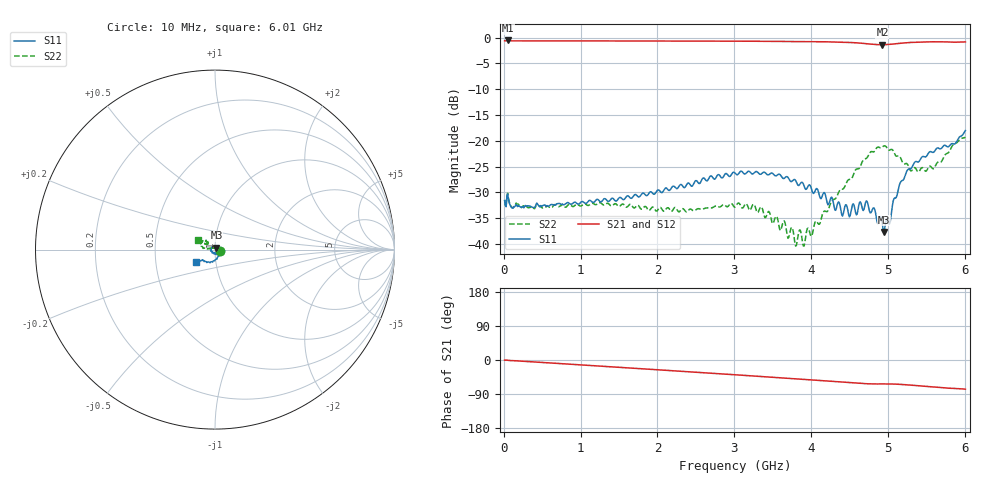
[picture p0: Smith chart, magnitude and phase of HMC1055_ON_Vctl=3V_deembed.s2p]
! Device:	HMC1055
! Description:	GaAs MMIC SPST Switch
! Package:	LP2 8 pin 2x2 mm QFN Plastic Package
! Frequency:	0.5 -  4 GHz
! Ports:
! RF1 = Port 1
! RF2 = Port 2
! State: ON
! Supply Votage: Vdd = 3 V
! ControlVoltage: Vctl = 3 V
! Data:	Data was collected using a calibrated network analyzer with AFR software.
!	Fixtures were calculated using AFR and fixturing was applied to collect
!	this Deembedded  S Parameter data of HMC1055.
!  The reference plane is the edge of the package pin.
! Note:	Analog Devices supplies this data as a sample of measured data at the package pin
!	for this product.  Your particular data for this product may vary.
!	Data was taken at 25 degrees C.
!	Analog Devices reserves the right to change this data at anytime.
# Hz S  dB  R 50
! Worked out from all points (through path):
!   601 points, 10 MHz to 6.01 GHz, reference 50 ohm
!   highest |S21| = -0.53 dB at 50 MHz (marker M1); lowest = -1.4 dB at 4.93 GHz (marker M2)
!   group delay of S21, straight-line fit = 35.6 ps
!   lowest |S11| = -37.6 dB at 4.95 GHz (marker M3), VSWR 1.03, Z = 50.8 + j1.04 ohm
!   |S11| at or under -10 dB: start of sweep to end of sweep
!   |S22| runs from -40.4 to -19.3 dB; largest |S21 - S12| = 0.004
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1e7  -31.59 -13.5  -0.60 -0.4  -0.59 -0.5  -31.46 -13.6
5e7  -30.32 -7.0  -0.53 -0.8  -0.53 -0.9  -30.17 -6.4
1.2e8  -33.06 -5.1  -0.61 -1.6  -0.61 -1.6  -32.97 -3.3
1.01e9  -31.82 -0.1  -0.62 -13.0  -0.62 -13.0  -32.61 -0.2
2.01e9  -29.50 2.5  -0.64 -25.9  -0.64 -26.0  -33.29 -1.9
3.01e9  -26.22 -9.2  -0.68 -39.0  -0.66 -39.1  -32.86 20.6
3.35e9  -26.44 -18.2  -0.69 -43.5  -0.68 -43.7  -32.78 35.3
3.65e9  -27.29 -27.0  -0.71 -47.6  -0.70 -47.8  -35.52 59.1
3.7e9  -27.08 -25.6  -0.72 -48.3  -0.71 -48.5  -38.90 61.8
3.75e9  -27.87 -31.9  -0.72 -49.0  -0.72 -49.2  -36.76 75.5
3.8e9  -27.71 -30.1  -0.73 -49.7  -0.72 -49.9  -40.43 82.3
4.01e9  -29.54 -41.5  -0.76 -52.6  -0.76 -52.8  -38.41 135.5
4.41e9  -34.58 -99.2  -0.87 -58.4  -0.87 -58.6  -29.38 173.6
4.73e9  -31.75 166.6  -1.18 -62.7  -1.17 -62.9  -23.26 169.3
4.93e9  -36.16 81.0  -1.38 -63.2  -1.37 -63.4  -21.16 149.3
4.95e9  -37.65 51.1  -1.36 -63.1  -1.35 -63.3  -20.99 146.8
5.01e9  -35.67 12.8  -1.30 -63.2  -1.29 -63.3  -21.78 142.2
5.16e9  -28.17 -56.6  -1.09 -64.3  -1.08 -64.4  -23.13 135.7
5.26e9  -25.59 -77.2  -0.96 -65.7  -0.95 -65.8  -24.62 137.5
5.6e9  -22.16 -117.4  -0.79 -71.1  -0.78 -71.3  -25.37 145.9
5.87e9  -20.60 -139.6  -0.87 -75.2  -0.86 -75.4  -20.53 151.6
6.01e9  -17.99 -148.2  -0.82 -77.0  -0.81 -77.2  -19.28 148.9
